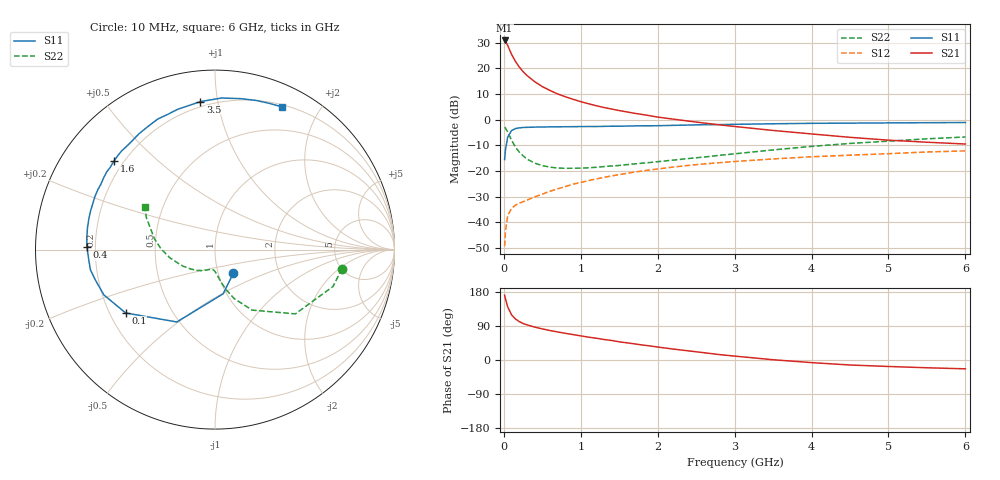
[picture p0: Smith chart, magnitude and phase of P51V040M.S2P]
! SIEMENS Small Signal Semiconductors
! BFP183
! Si NPN RF Bipolar Junction Transistor in SOT143
! VCE = 1 V  IC = 40 mA
! Common Emitter S-Parameters:  March  1996
# GHz  S  MA  R  50
!  f  S11  S21  S12  S22
! GHz  MAG  ANG  MAG  ANG  MAG  ANG  MAG  ANG
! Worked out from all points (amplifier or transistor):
!   36 points, 10 MHz to 6 GHz, reference 50 ohm
!   highest |S21| = 30.9 dB at 10 MHz (marker M1)
!   |S21| within 3 dB of that: start of sweep to 65.35 MHz
!   unconditionally stable (mu >= 1): start of sweep to 23.48 MHz; 207.7 MHz to end of sweep
!   at 250 MHz: K = 1.11, MAG = 23.3 dB, |S12| = -32.0 dB
!   at 1.4 GHz: K = 1.77, MAG = 8.0 dB, |S12| = -22.0 dB
!   at 6 GHz: K = 1.42, MAG = -2.5 dB, |S12| = -12.2 dB
!   S11 on the Smith chart (normalised r, x): 10 MHz: 1.18, -0.32; 100 MHz: 0.26, -0.30; 400 MHz: 0.17, +0.01; 1.6 GHz: 0.16, +0.37; 3.5 GHz: 0.17, +0.89; 6 GHz: 0.22, +1.55
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0.01  0.1661 -51.7  34.94 170.9  0.0034 72.5  0.7152 -8.6
0.02  0.2502 -79.5  33.86 162.2  0.0065 68.2  0.6887 -17.4
0.05  0.4559 -117.8  27.94 140.3  0.0134 58.2  0.573 -38.7
0.1  0.6106 -144.7  18.79 119.4  0.0186 44.3  0.3953 -58.5
0.15  0.6685 -157.8  13.69 108.4  0.0214 42.1  0.2923 -68.7
0.2  0.6873 -165.6  10.64 101.4  0.0234 41.8  0.2334 -74.2
0.25  0.7031 -170.7  8.633 96.4  0.025 43.4  0.1968 -78.0
0.3  0.7051 -174.9  7.256 92.8  0.0269 45.5  0.1705 -81.0
0.4  0.714 179.0  5.505 86.9  0.031 49.6  0.1417 -85.2
0.5  0.7174 174.1  4.399 82.1  0.0351 51.1  0.1266 -88.5
0.6  0.721 170.2  3.7 77.8  0.0401 54.2  0.1181 -91.7
0.7  0.7237 166.2  3.16 74.0  0.0446 56.1  0.1136 -94.7
0.9  0.7273 159.7  2.488 67.1  0.0551 57.1  0.1126 -99.7
1.1  0.7332 153.0  2.039 60.3  0.0646 57.3  0.1149 -105.2
1.3  0.7378 147.4  1.723 54.2  0.0745 56.8  0.1211 -110.6
1.6  0.7484 138.8  1.412 45.3  0.0896 54.8  0.1323 -118.6
2.2  0.7719 123.3  1.022 28.9  0.1187 49.1  0.1621 -136.2
2.8  0.7983 109.1  0.791 14.3  0.1442 42.4  0.2007 -152.6
3.5  0.8286 95.6  0.614 0.7  0.1709 34.8  0.2564 -169.9
4.5  0.8532 80.3  0.451 -13.2  0.2022 24.0  0.3431 169.8
5.5  0.8695 69.5  0.362 -20.5  0.2336 14.5  0.4219 155.0
6  0.8778 65.0  0.334 -23.3  0.2452 9.3  0.458 148.5
